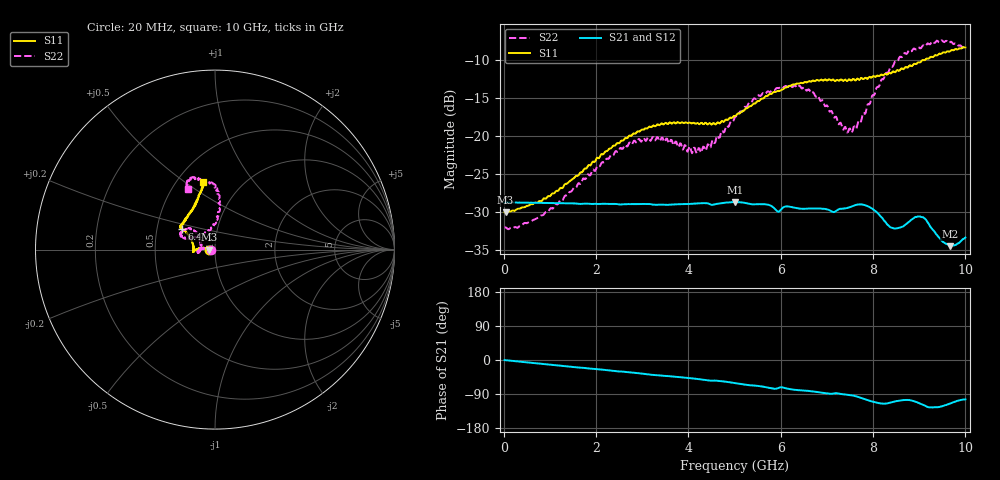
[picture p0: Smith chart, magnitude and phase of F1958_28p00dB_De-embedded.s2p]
! Integrated Device Technology
! Corporate Headquarters
! 6024 Silver Creek Valley Road
! San Jose, CA 95138  USA
! Phone:  1-408-284-8200
! Toll Free:  1-800-223-1366
! Webpage:  http://www.idt.com/
! Timing and RF Division
! 515 Groton Road, Suite 102
! Westford, MA 01886-6024
! Device:  F1958
! Description: 7-bit 0.25 dB Digital Step Attenuator
! Frequency:  0.001 -  6.000 GHz
! Package:  4x4 mm Thin QFN Plastic Package: 24 pin
! Ports:  2 RF, 12 DC
!  Pin  1  = D0
!  Pin  2  = VDD
!  Pin  3  = VMODE
!  Pin  4  = GND
!  Pin  5  = RF1  =  Port 1
!  Pin  6  = GND
!  Pin  7  = GND
!  Pin  8  = GND
!  Pin  9  = GND
!  Pin 10  = GND
!  Pin 11  = GND
!  Pin 12  = GND
!  Pin 13  = GND
!  Pin 14  = RF2  =  Port 2
!  Pin 15  = GND
!  Pin 16  = LE
!  Pin 17  = CLK
!  Pin 18  = DATA
!  Pin 19  = D6
!  Pin 20  = D5
!  Pin 21  = D4
!  Pin 22  = D3
!  Pin 23  = D2
!  Pin 24  = D1
! State:  112
! Atten State:  28.00 dB
! Voltage:  +3.30 Volts
! Current:  0.258 mA
! Data:  The device was measured on a F1958 evaluation board which has
!  individual transmission lines to the RF pins.  Data was collected
!  using a calibrated network analyzer.  The evaluation board was
!  de-embedded using Automatic Fixture Removal (AFR).
!  The reference plane is the edge of the package pin.
! Misc:
!  Action Tracker AT0419
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# GHz S dB R 50
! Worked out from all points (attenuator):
!   500 points, 20 MHz to 10 GHz, reference 50 ohm
!   highest |S21| = -28.72 dB at 5.02 GHz (marker M1); lowest = -34.5 dB at 9.66 GHz (marker M2)
!   lowest |S11| = -30.1 dB at 40 MHz (marker M3), VSWR 1.06, Z = 47 - j0.0447 ohm
!   |S11| at or under -10 dB: start of sweep to 9.13 GHz
!   |S22| runs from -32.3 to -7.5 dB; largest |S21 - S12| = 0.00028
!   S11 on the Smith chart (normalised r, x): 20 MHz: 0.94, -0.00; 6.4 GHz: 0.67, +0.16; 10 GHz: 0.67, +0.59
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0.02  -30.04 -178.9  -28.79 -0.2  -28.77 -0.2  -32.07 -178.9
0.04  -30.07 -179.1  -28.78 -0.4  -28.78 -0.4  -32.03 -178.4
0.84  -28.45 171.0  -28.82 -10.3  -28.82 -10.2  -30.46 172.0
1.7  -24.79 171.1  -28.94 -20.4  -28.94 -20.4  -25.89 171.1
2.62  -20.38 177.1  -29.00 -31.2  -28.98 -31.3  -21.24 -179.6
3.36  -18.59 -175.5  -29.07 -40.4  -29.07 -40.6  -20.53 -169.3
4.24  -18.49 -178.8  -28.89 -50.6  -28.89 -50.7  -21.65 169.0
4.5  -18.54 175.3  -29.08 -54.5  -29.09 -54.6  -21.02 151.4
5.02  -17.40 161.0  -28.72 -61.1  -28.74 -61.1  -17.42 138.2
5.58  -15.14 150.7  -29.00 -69.6  -29.01 -69.5  -14.67 140.0
5.94  -14.11 148.5  -29.98 -74.4  -29.99 -74.4  -13.74 148.8
6.4  -13.16 148.0  -29.57 -79.7  -29.58 -79.7  -13.44 155.9
6.68  -12.80 146.8  -29.55 -82.7  -29.56 -82.6  -14.37 158.0
7.14  -12.61 142.9  -30.03 -88.8  -30.05 -88.6  -17.41 152.4
7.5  -12.62 138.4  -29.39 -92.4  -29.40 -92.4  -19.04 120.3
7.68  -12.58 135.5  -29.04 -97.6  -29.03 -97.6  -18.11 99.9
7.9  -12.38 129.0  -29.30 -106.6  -29.30 -106.6  -15.80 89.5
8.34  -11.75 118.9  -31.83 -113.8  -31.83 -113.8  -11.55 84.1
8.66  -11.26 113.2  -31.90 -105.7  -31.87 -105.9  -9.31 87.9
9.06  -10.10 106.8  -30.70 -117.0  -30.71 -117.3  -8.29 97.8
9.66  -8.93 100.7  -34.51 -115.4  -34.43 -115.2  -7.74 110.4
10  -8.41 99.8  -33.38 -103.8  -33.43 -103.6  -8.60 114.2
